| IBIS file stm32l0_71_72_73_81_82_83_lqfp64.ibs
| Created by s2ibis version 1.1 (customized version)
| North Carolina State University, ERL, 2006
[IBIS ver] 4.2
[File name] stm32l0_71_72_73_81_82_83_lqfp64.ibs
[File Rev] 1.0
[Date]  14-03-2016
[Source] Data Created at STMicroelectronics
[Notes]  File originated from ELDO simulations.
[Disclaimer]  This information is for modeling purpose only and is
   not guaranted. The information is subject to change without
   notice.
[Copyright] Copyright 2016 STMicroelectronics Inc.
|   Component stm32l0_71_72_73_81_82_83_lqfp64
[Component] stm32l0_71_72_73_81_82_83_lqfp64
[Manufacturer] STMicroelectronics
[Package]
| variable   typ   min   max
R_pkg   0.0   0.0   0.0
L_pkg   0.0H   0.0H   0.0H
C_pkg   0.0F   0.0F   0.0F
[Pin]  signal_name   model_name   R_pin   L_pin   C_pin
1 VLCD POWER   68.980E-3   4.220E-9   120.000E-15
2 PC13 io8p_wsudq_ls_ft_v33   63.756E-3   3.679E-9   93.469E-15
3 PC14-OSC32_IN io8p_wsudq_ls_ft_v33   59.336E-3   3.221E-9   71.020E-15
4 PC15-OSC32_OUT io8p_sudq_ls_tc_esdft 55.719E-3   2.846E-9   52.653E-15
5 PH0-OSC_IN io8p_sudq_ls_tc_esdft   52.907E-3   2.555E-9   38.367E-15
6 PH1-OSC_OUT io8p_sudq_ls_tc_esdft   50.897E-3   2.347E-9   28.163E-15
7 NRST ioreset_ft_v33   49.692E-3   2.222E-9   22.041E-15
8 PC0 io8p_sudq_lcd4_i2cin_ls_ft   49.290E-3   2.180E-9   20.000E-15
9 PC1 io8p_sudq_lcd4_i2cin_ls_ft   49.290E-3   2.180E-9   20.000E-15
10 PC2 io8p_wsudq_lcd4_ls_ft   49.692E-3   2.222E-9   22.041E-15
11 PC3 io8p_wsudq_lcd4_ls_ft   50.897E-3   2.347E-9   28.163E-15
12 VSSA GND   52.907E-3   2.555E-9   38.367E-15
13 VDDA POWER   55.719E-3   2.846E-9   52.653E-15
14 PA0 io8p_wsudq_ls_ft_v33   59.336E-3   3.221E-9   71.020E-15
15 PA1 io8p_wsudq_lcd4_ls_ft  63.756E-3   3.679E-9   93.469E-15
16 PA2 io8p_wsudq_lcd4_ls_ft  68.980E-3   4.220E-9   120.000E-15
17 PA3 io8p_wsudq_lcd4_ls_ft  68.980E-3   4.220E-9   120.000E-15
18 VSS GND   63.756E-3   3.679E-9   93.469E-15
19 VDD POWER   59.336E-3   3.221E-9   71.020E-15
20 PA4 io8p_wsudq_i2cin_ls_ft 55.719E-3   2.846E-9   52.653E-15
21 PA5 io8p_wsudq_i2cin_ls_ft 52.907E-3   2.555E-9   38.367E-15
22 PA6 io8p_wsudq_lcd4_ls_ft  50.897E-3   2.347E-9   28.163E-15
23 PA7 io8p_wsudq_lcd4_ls_ft  49.692E-3   2.222E-9   22.041E-15
24 PC4 io8p_wsudq_lcd4_ls_ft  49.290E-3   2.180E-9   20.000E-15
25 PC5 io8p_wsudq_lcd4_ls_ft  49.290E-3   2.180E-9   20.000E-15
26 PB0 io8p_wsudq_lcd4_ls_ft  49.692E-3   2.222E-9   22.041E-15
27 PB1 io8p_wsudq_lcd4_ls_ft  50.897E-3   2.347E-9   28.163E-15
28 PB2 io8p_wsudq_lcd4_ls_ft  52.907E-3   2.555E-9   38.367E-15
29 PB10 io8p_sudq_lcd4_i2cin_ls_ft   55.719E-3   2.846E-9   52.653E-15
30 PB11 io8p_sudq_lcd4_i2cin_ls_ft   59.336E-3   3.221E-9   71.020E-15
31 VSS GND   63.756E-3   3.679E-9   93.469E-15
32 VDD POWER   68.980E-3   4.220E-9   120.000E-15
33 PB12 io8p_wsudq_lcd4_ls_ft 68.980E-3   4.220E-9   120.000E-15
34 PB13 io8p_sudq_lcd4_i2cin_ls_ft   63.756E-3   3.679E-9   93.469E-15
35 PB14 io8p_sudq_lcd4_i2cin_ls_ft   59.336E-3   3.221E-9   71.020E-15
36 PB15 io8p_wsudq_lcd4_ls_ft   55.719E-3   2.846E-9   52.653E-15
37 PC6 io8p_wsudq_lcd4_ls_ft   52.907E-3   2.555E-9   38.367E-15
38 PC7 io8p_wsudq_lcd4_ls_ft   50.897E-3   2.347E-9   28.163E-15
39 PC8 io8p_wsudq_lcd4_ls_ft   49.692E-3   2.222E-9   22.041E-15
40 PC9 io8p_sudq_lcd4_i2cin_ls_ft   49.290E-3   2.180E-9   20.000E-15
41 PA8 io8p_sudq_lcd4_i2cin_ls_ft   49.290E-3   2.180E-9   20.000E-15
42 PA9 io8p_sudq_lcd4_i2cin_ls_ft   49.692E-3   2.222E-9   22.041E-15
43 PA10 io8p_sudq_lcd4_i2cin_ls_ft   50.897E-3   2.347E-9   28.163E-15
44 PA11 io8usb_ls_ft   52.907E-3   2.555E-9   38.367E-15
45 PA12 io8usb_ls_ft   55.719E-3   2.846E-9   52.653E-15
46 PA13 io8p_sudq_ls_ft   59.336E-3   3.221E-9   71.020E-15
47 VSS GND   63.756E-3   3.679E-9   93.469E-15
48 VDD_USB POWER   68.980E-3   4.220E-9   120.000E-15
49 PA14 io8p_sudq_ls_ft   68.980E-3   4.220E-9   120.000E-15
50 PA15 io8p_wsudq_lcd4_ls_ft   63.756E-3   3.679E-9   93.469E-15
51 PC10 io8p_wsudq_lcd4_ls_ft   59.336E-3   3.221E-9   71.020E-15
52 PC11 io8p_wsudq_lcd4_ls_ft   55.719E-3   2.846E-9   52.653E-15
53 PC12 io8p_wsudq_lcd4_ls_ft   52.907E-3   2.555E-9   38.367E-15
54 PD2 io8p_wsudq_lcd4_ls_ft   50.897E-3   2.347E-9   28.163E-15
55 PB3 io8p_wsudq_lcd4_ls_ft   49.692E-3   2.222E-9   22.041E-15
56 PB4 io8p_sudq_lcd4_i2cin_ls_ft 49.290E-3   2.180E-9   20.000E-15
57 PB5 io8p_wsudq_lcd4_ls_ft   49.290E-3   2.180E-9   20.000E-15
58 PB6 io8p_wsudq_i2cin_ls_ft   49.692E-3   2.222E-9   22.041E-15
59 PB7 io8p_wsudq_i2cin_ls_ft   50.897E-3   2.347E-9   28.163E-15
60 BOOT0 vpp_test_hv  52.907E-3   2.555E-9   38.367E-15
61 PB8 io8p_sudq_lcd4_i2cin_ls_ft   55.719E-3   2.846E-9   52.653E-15
62 PB9 io8p_sudq_lcd4_i2cin_ls_ft   59.336E-3   3.221E-9   71.020E-15
63 VSS GND   63.756E-3   3.679E-9   93.469E-15
64 VDD POWER   68.980E-3   4.220E-9   120.000E-15
[Model Selector] io8p_sudq_ls_ft
io8p00_sudq_ls_ft_pd_lv  "SPEED00 1P8V, PD=40kOhm"
io8p00_sudq_ls_ft_pu_lv  "SPEED00 1P8V, PU=40kOhm"
io8p00_sudq_ls_ft_lv  "SPEED00 1P8V"
io8p01_sudq_ls_ft_pd_lv  "SPEED01 1P8V, PD=40kOhm"
io8p01_sudq_ls_ft_pu_lv  "SPEED01 1P8V, PU=40kOhm"
io8p01_sudq_ls_ft_lv  "SPEED01 1P8V"
io8p10_sudq_ls_ft_pd_lv  "SPEED10 1P8V, PD=40kOhm"
io8p10_sudq_ls_ft_pu_lv  "SPEED10 1P8V, PU=40kOhm"
io8p10_sudq_ls_ft_lv  "SPEED10 1P8V"
io8p11_sudq_ls_ft_pd_lv  "SPEED11 1P8V, PD=40kOhm"
io8p11_sudq_ls_ft_pu_lv  "SPEED11 1P8V, PU=40kOhm"
io8p11_sudq_ls_ft_lv  "SPEED11 1P8V"
io8p00_sudq_ls_ft_pd  "SPEED00, PD=40kOhm"
io8p00_sudq_ls_ft_pu  "SPEED00, PU=40kOhm"
io8p00_sudq_ls_ft  "SPEED00"
io8p01_sudq_ls_ft_pd  "SPEED01, PD=40kOhm"
io8p01_sudq_ls_ft_pu  "SPEED01, PU=40kOhm"
io8p01_sudq_ls_ft  "SPEED01"
io8p10_sudq_ls_ft_pd  "SPEED10, PD=40kOhm"
io8p10_sudq_ls_ft_pu  "SPEED10, PU=40kOhm"
io8p10_sudq_ls_ft  "SPEED10"
io8p11_sudq_ls_ft_pd  "SPEED11, PD=40kOhm"
io8p11_sudq_ls_ft_pu  "SPEED11, PU=40kOhm"
io8p11_sudq_ls_ft  "SPEED11"
[Model Selector] io8p_sudq_ls_tc_esdft
io8p00_sudq_ls_tc_esdft_pd_lv  "SPEED00 1P8V, PD=40kOhm"
io8p00_sudq_ls_tc_esdft_pu_lv  "SPEED00 1P8V, PU=40kOhm"
io8p00_sudq_ls_tc_esdft_lv  "SPEED00 1P8V"
io8p01_sudq_ls_tc_esdft_pd_lv  "SPEED01 1P8V, PD=40kOhm"
io8p01_sudq_ls_tc_esdft_pu_lv  "SPEED01 1P8V, PU=40kOhm"
io8p01_sudq_ls_tc_esdft_lv  "SPEED01 1P8V"
io8p10_sudq_ls_tc_esdft_pd_lv  "SPEED10 1P8V, PD=40kOhm"
io8p10_sudq_ls_tc_esdft_pu_lv  "SPEED10 1P8V, PU=40kOhm"
io8p10_sudq_ls_tc_esdft_lv  "SPEED10 1P8V"
io8p11_sudq_ls_tc_esdft_pd_lv  "SPEED11 1P8V, PD=40kOhm"
io8p11_sudq_ls_tc_esdft_pu_lv  "SPEED11 1P8V, PU=40kOhm"
io8p11_sudq_ls_tc_esdft_lv  "SPEED11 1P8V"
io8p00_sudq_ls_tc_esdft_pd  "SPEED00, PD=40kOhm"
io8p00_sudq_ls_tc_esdft_pu  "SPEED00, PU=40kOhm"
io8p00_sudq_ls_tc_esdft  "SPEED00"
io8p01_sudq_ls_tc_esdft_pd  "SPEED01, PD=40kOhm"
io8p01_sudq_ls_tc_esdft_pu  "SPEED01, PU=40kOhm"
io8p01_sudq_ls_tc_esdft  "SPEED01"
io8p10_sudq_ls_tc_esdft_pd  "SPEED10, PD=40kOhm"
io8p10_sudq_ls_tc_esdft_pu  "SPEED10, PU=40kOhm"
io8p10_sudq_ls_tc_esdft  "SPEED10"
io8p11_sudq_ls_tc_esdft_pd  "SPEED11, PD=40kOhm"
io8p11_sudq_ls_tc_esdft_pu  "SPEED11, PU=40kOhm"
io8p11_sudq_ls_tc_esdft  "SPEED11"
[Model Selector] io8p_wsudq_i2cin_ls_ft
io8p00_wsudq_i2cin_ls_ft_pd_lv  "SPEED00 1P8V, PD=40kOhm"
io8p00_wsudq_i2cin_ls_ft_pu_lv  "SPEED00 1P8V, PU=40kOhm"
io8p00_wsudq_i2cin_ls_ft_lv  "SPEED00 1P8V"
io8p01_wsudq_i2cin_ls_ft_pd_lv  "SPEED01 1P8V, PD=40kOhm"
io8p01_wsudq_i2cin_ls_ft_pu_lv  "SPEED01 1P8V, PU=40kOhm"
io8p01_wsudq_i2cin_ls_ft_lv  "SPEED01 1P8V"
io8p10_wsudq_i2cin_ls_ft_pd_lv  "SPEED10 1P8V, PD=40kOhm"
io8p10_wsudq_i2cin_ls_ft_pu_lv  "SPEED10 1P8V, PU=40kOhm"
io8p10_wsudq_i2cin_ls_ft_lv  "SPEED10 1P8V"
io8p11_wsudq_i2cin_ls_ft_pd_lv  "SPEED11 1P8V, PD=40kOhm"
io8p11_wsudq_i2cin_ls_ft_pu_lv  "SPEED11 1P8V, PU=40kOhm"
io8p11_wsudq_i2cin_ls_ft_lv  "SPEED11 1P8V"
io8p00_wsudq_i2cin_ls_ft_pd  "SPEED00, PD=40kOhm"
io8p00_wsudq_i2cin_ls_ft_pu  "SPEED00, PU=40kOhm"
io8p00_wsudq_i2cin_ls_ft  "SPEED00"
io8p01_wsudq_i2cin_ls_ft_pd  "SPEED01, PD=40kOhm"
io8p01_wsudq_i2cin_ls_ft_pu  "SPEED01, PU=40kOhm"
io8p01_wsudq_i2cin_ls_ft  "SPEED01"
io8p10_wsudq_i2cin_ls_ft_pd  "SPEED10, PD=40kOhm"
io8p10_wsudq_i2cin_ls_ft_pu  "SPEED10, PU=40kOhm"
io8p10_wsudq_i2cin_ls_ft  "SPEED10"
io8p11_wsudq_i2cin_ls_ft_pd  "SPEED11, PD=40kOhm"
io8p11_wsudq_i2cin_ls_ft_pu  "SPEED11, PU=40kOhm"
io8p11_wsudq_i2cin_ls_ft  "SPEED11"
[Model Selector] io8p_wsudq_lcd4_ls_ft
io8p00_wsudq_lcd4_ls_ft_pd_lv  "SPEED00 1P8V, PD=40kOhm"
io8p00_wsudq_lcd4_ls_ft_pu_lv  "SPEED00 1P8V, PU=40kOhm"
io8p00_wsudq_lcd4_ls_ft_lv  "SPEED00 1P8V"
io8p01_wsudq_lcd4_ls_ft_pd_lv  "SPEED01 1P8V, PD=40kOhm"
io8p01_wsudq_lcd4_ls_ft_pu_lv  "SPEED01 1P8V, PU=40kOhm"
io8p01_wsudq_lcd4_ls_ft_lv  "SPEED01 1P8V"
io8p10_wsudq_lcd4_ls_ft_pd_lv  "SPEED10 1P8V, PD=40kOhm"
io8p10_wsudq_lcd4_ls_ft_pu_lv  "SPEED10 1P8V, PU=40kOhm"
io8p10_wsudq_lcd4_ls_ft_lv  "SPEED10 1P8V"
io8p11_wsudq_lcd4_ls_ft_pd_lv  "SPEED11 1P8V, PD=40kOhm"
io8p11_wsudq_lcd4_ls_ft_pu_lv  "SPEED11 1P8V, PU=40kOhm"
io8p11_wsudq_lcd4_ls_ft_lv  "SPEED11 1P8V"
io8p00_wsudq_lcd4_ls_ft_pd  "SPEED00, PD=40kOhm"
io8p00_wsudq_lcd4_ls_ft_pu  "SPEED00, PU=40kOhm"
io8p00_wsudq_lcd4_ls_ft  "SPEED00"
io8p01_wsudq_lcd4_ls_ft_pd  "SPEED01, PD=40kOhm"
io8p01_wsudq_lcd4_ls_ft_pu  "SPEED01, PU=40kOhm"
io8p01_wsudq_lcd4_ls_ft  "SPEED01"
io8p10_wsudq_lcd4_ls_ft_pd  "SPEED10, PD=40kOhm"
io8p10_wsudq_lcd4_ls_ft_pu  "SPEED10, PU=40kOhm"
io8p10_wsudq_lcd4_ls_ft  "SPEED10"
io8p11_wsudq_lcd4_ls_ft_pd  "SPEED11, PD=40kOhm"
io8p11_wsudq_lcd4_ls_ft_pu  "SPEED11, PU=40kOhm"
io8p11_wsudq_lcd4_ls_ft  "SPEED11"
[Model Selector] io8p_wsudq_ls_ft_v33
io8p00_wsudq_ls_ft_v33_pd_lv  "SPEED00 1P8V, PD=40kOhm"
io8p00_wsudq_ls_ft_v33_pu_lv  "SPEED00 1P8V, PU=40kOhm"
io8p00_wsudq_ls_ft_v33_lv  "SPEED00 1P8V"
io8p01_wsudq_ls_ft_v33_pd_lv  "SPEED01 1P8V, PD=40kOhm"
io8p01_wsudq_ls_ft_v33_pu_lv  "SPEED01 1P8V, PU=40kOhm"
io8p01_wsudq_ls_ft_v33_lv  "SPEED01 1P8V"
io8p10_wsudq_ls_ft_v33_pd_lv  "SPEED10 1P8V, PD=40kOhm"
io8p10_wsudq_ls_ft_v33_pu_lv  "SPEED10 1P8V, PU=40kOhm"
io8p10_wsudq_ls_ft_v33_lv  "SPEED10 1P8V"
io8p11_wsudq_ls_ft_v33_pd_lv  "SPEED11 1P8V, PD=40kOhm"
io8p11_wsudq_ls_ft_v33_pu_lv  "SPEED11 1P8V, PU=40kOhm"
io8p11_wsudq_ls_ft_v33_lv  "SPEED11 1P8V"
io8p00_wsudq_ls_ft_v33_pd  "SPEED00, PD=40kOhm"
io8p00_wsudq_ls_ft_v33_pu  "SPEED00, PU=40kOhm"
io8p00_wsudq_ls_ft_v33  "SPEED00"
io8p01_wsudq_ls_ft_v33_pd  "SPEED01, PD=40kOhm"
io8p01_wsudq_ls_ft_v33_pu  "SPEED01, PU=40kOhm"
io8p01_wsudq_ls_ft_v33  "SPEED01"
io8p10_wsudq_ls_ft_v33_pd  "SPEED10, PD=40kOhm"
io8p10_wsudq_ls_ft_v33_pu  "SPEED10, PU=40kOhm"
io8p10_wsudq_ls_ft_v33  "SPEED10"
io8p11_wsudq_ls_ft_v33_pd  "SPEED11, PD=40kOhm"
io8p11_wsudq_ls_ft_v33_pu  "SPEED11, PU=40kOhm"
io8p11_wsudq_ls_ft_v33  "SPEED11"
[Model Selector] vpp_test_hv
vpp_test_hv_2p4  "Input Buffer 1P65V"
vpp_test_hv_3p3  "Input Buffer"
[Model Selector] io8usb_ls_ft
io8usb_ls_ft_dpdn_pu  "HS USB DP/DN IO + PU=1.2kOhm"
io8usb_ls_ft_dpdn  "HS USB DP/DN IO"
io8p00_ls_ft_pd_lv  "SPEED00 1P8V, PD=40kOhm"
io8p00_ls_ft_pu_lv  "SPEED00 1P8V, PU=40kOhm"
io8p00_ls_ft_lv  "SPEED00 1P8V"
io8p01_ls_ft_pd_lv  "SPEED01 1P8V, PD=40kOhm"
io8p01_ls_ft_pu_lv  "SPEED01 1P8V, PU=40kOhm"
io8p01_ls_ft_lv  "SPEED01 1P8V"
io8p10_ls_ft_pd_lv  "SPEED10 1P8V, PD=40kOhm"
io8p10_ls_ft_pu_lv  "SPEED10 1P8V, PU=40kOhm"
io8p10_ls_ft_lv  "SPEED10 1P8V"
io8p11_ls_ft_pd_lv  "SPEED11 1P8V, PD=40kOhm"
io8p11_ls_ft_pu_lv  "SPEED11 1P8V, PU=40kOhm"
io8p11_ls_ft_lv  "SPEED11 1P8V"
io8p00_ls_ft_pd  "SPEED00, PD=40kOhm"
io8p00_ls_ft_pu  "SPEED00, PU=40kOhm"
io8p00_ls_ft  "SPEED00"
io8p01_ls_ft_pd  "SPEED01, PD=40kOhm"
io8p01_ls_ft_pu  "SPEED01, PU=40kOhm"
io8p01_ls_ft  "SPEED01"
io8p10_ls_ft_pd  "SPEED10, PD=40kOhm"
io8p10_ls_ft_pu  "SPEED10, PU=40kOhm"
io8p10_ls_ft  "SPEED10"
io8p11_ls_ft_pd  "SPEED11, PD=40kOhm"
io8p11_ls_ft_pu  "SPEED11, PU=40kOhm"
io8p11_ls_ft  "SPEED11"
[Model Selector] io8p_sudq_lcd4_i2cin_ls_ft
io8p00_sudq_lcd4_i2cin_ls_ft_pd_lv  "SPEED00 1P8V, PD=40kOhm"
io8p00_sudq_lcd4_i2cin_ls_ft_pu_lv  "SPEED00 1P8V, PU=40kOhm"
io8p00_sudq_lcd4_i2cin_ls_ft_lv  "SPEED00 1P8V"
io8p01_sudq_lcd4_i2cin_ls_ft_pd_lv  "SPEED01 1P8V, PD=40kOhm"
io8p01_sudq_lcd4_i2cin_ls_ft_pu_lv  "SPEED01 1P8V, PU=40kOhm"
io8p01_sudq_lcd4_i2cin_ls_ft_lv  "SPEED01 1P8V"
io8p10_sudq_lcd4_i2cin_ls_ft_pd_lv  "SPEED10 1P8V, PD=40kOhm"
io8p10_sudq_lcd4_i2cin_ls_ft_pu_lv  "SPEED10 1P8V, PU=40kOhm"
io8p10_sudq_lcd4_i2cin_ls_ft_lv  "SPEED10 1P8V"
io8p11_sudq_lcd4_i2cin_ls_ft_pd_lv  "SPEED11 1P8V, PD=40kOhm"
io8p11_sudq_lcd4_i2cin_ls_ft_pu_lv  "SPEED11 1P8V, PU=40kOhm"
io8p11_sudq_lcd4_i2cin_ls_ft_lv  "SPEED11 1P8V"
io8p00_sudq_lcd4_i2cin_ls_ft_pd  "SPEED00, PD=40kOhm"
io8p00_sudq_lcd4_i2cin_ls_ft_pu  "SPEED00, PU=40kOhm"
io8p00_sudq_lcd4_i2cin_ls_ft  "SPEED00"
io8p01_sudq_lcd4_i2cin_ls_ft_pd  "SPEED01, PD=40kOhm"
io8p01_sudq_lcd4_i2cin_ls_ft_pu  "SPEED01, PU=40kOhm"
io8p01_sudq_lcd4_i2cin_ls_ft  "SPEED01"
io8p10_sudq_lcd4_i2cin_ls_ft_pd  "SPEED10, PD=40kOhm"
io8p10_sudq_lcd4_i2cin_ls_ft_pu  "SPEED10, PU=40kOhm"
io8p10_sudq_lcd4_i2cin_ls_ft  "SPEED10"
io8p11_sudq_lcd4_i2cin_ls_ft_pd  "SPEED11, PD=40kOhm"
io8p11_sudq_lcd4_i2cin_ls_ft_pu  "SPEED11, PU=40kOhm"
io8p11_sudq_lcd4_i2cin_ls_ft  "SPEED11"
[Model Selector] ioreset_ft_v33
ioreset_ft_v33_pu_lv  "ioreset 1P8V + PU=40kOhm"
ioreset_ft_v33_nopu_lv  "ioreset 1P8V"
ioreset_ft_v33_pu  "ioreset + PU=40kOhm"
ioreset_ft_v33_nopu  "ioreset"
| Models and submodels in the file (176): io8p00_sudq_ls_ft_pd_lv (I/O), io8p00_sudq_ls_ft_pu_lv (I/O), io8p00_sudq_ls_ft_lv (I/O), io8p01_sudq_ls_ft_pd_lv (I/O), io8p01_sudq_ls_ft_pu_lv (I/O), io8p01_sudq_ls_ft_lv (I/O), io8p10_sudq_ls_ft_pd_lv (I/O), io8p10_sudq_ls_ft_pu_lv (I/O), io8p10_sudq_ls_ft_lv (I/O), io8p11_sudq_ls_ft_pd_lv (I/O), io8p11_sudq_ls_ft_pu_lv (I/O), io8p11_sudq_ls_ft_lv (I/O), io8p00_sudq_ls_ft_pd (I/O), io8p00_sudq_ls_ft_pu (I/O), io8p00_sudq_ls_ft (I/O), io8p01_sudq_ls_ft_pd (I/O), io8p01_sudq_ls_ft_pu (I/O), io8p01_sudq_ls_ft (I/O), io8p10_sudq_ls_ft_pd (I/O), io8p10_sudq_ls_ft_pu (I/O), io8p10_sudq_ls_ft (I/O), io8p11_sudq_ls_ft_pd (I/O), io8p11_sudq_ls_ft_pu (I/O), io8p11_sudq_ls_ft (I/O), io8p00_sudq_ls_tc_esdft_pd_lv (I/O), io8p00_sudq_ls_tc_esdft_pu_lv (I/O), io8p00_sudq_ls_tc_esdft_lv (I/O), io8p01_sudq_ls_tc_esdft_pd_lv (I/O), io8p01_sudq_ls_tc_esdft_pu_lv (I/O), io8p01_sudq_ls_tc_esdft_lv (I/O), io8p10_sudq_ls_tc_esdft_pd_lv (I/O), io8p10_sudq_ls_tc_esdft_pu_lv (I/O), io8p10_sudq_ls_tc_esdft_lv (I/O), io8p11_sudq_ls_tc_esdft_pd_lv (I/O), io8p11_sudq_ls_tc_esdft_pu_lv (I/O), io8p11_sudq_ls_tc_esdft_lv (I/O), io8p00_sudq_ls_tc_esdft_pd (I/O), io8p00_sudq_ls_tc_esdft_pu (I/O), io8p00_sudq_ls_tc_esdft (I/O), io8p01_sudq_ls_tc_esdft_pd (I/O), io8p01_sudq_ls_tc_esdft_pu (I/O), io8p01_sudq_ls_tc_esdft (I/O), io8p10_sudq_ls_tc_esdft_pd (I/O), io8p10_sudq_ls_tc_esdft_pu (I/O), io8p10_sudq_ls_tc_esdft (I/O), io8p11_sudq_ls_tc_esdft_pd (I/O), io8p11_sudq_ls_tc_esdft_pu (I/O), io8p11_sudq_ls_tc_esdft (I/O), io8p00_wsudq_i2cin_ls_ft_pd_lv (I/O), io8p00_wsudq_i2cin_ls_ft_pu_lv (I/O), io8p00_wsudq_i2cin_ls_ft_lv (I/O), io8p01_wsudq_i2cin_ls_ft_pd_lv (I/O), io8p01_wsudq_i2cin_ls_ft_pu_lv (I/O), io8p01_wsudq_i2cin_ls_ft_lv (I/O), io8p10_wsudq_i2cin_ls_ft_pd_lv (I/O), io8p10_wsudq_i2cin_ls_ft_pu_lv (I/O), io8p10_wsudq_i2cin_ls_ft_lv (I/O), io8p11_wsudq_i2cin_ls_ft_pd_lv (I/O), io8p11_wsudq_i2cin_ls_ft_pu_lv (I/O), io8p11_wsudq_i2cin_ls_ft_lv (I/O), io8p00_wsudq_i2cin_ls_ft_pd (I/O), io8p00_wsudq_i2cin_ls_ft_pu (I/O), io8p00_wsudq_i2cin_ls_ft (I/O), io8p01_wsudq_i2cin_ls_ft_pd (I/O), io8p01_wsudq_i2cin_ls_ft_pu (I/O), io8p01_wsudq_i2cin_ls_ft (I/O), io8p10_wsudq_i2cin_ls_ft_pd (I/O), io8p10_wsudq_i2cin_ls_ft_pu (I/O), io8p10_wsudq_i2cin_ls_ft (I/O), io8p11_wsudq_i2cin_ls_ft_pd (I/O), io8p11_wsudq_i2cin_ls_ft_pu (I/O), io8p11_wsudq_i2cin_ls_ft (I/O), io8p00_wsudq_lcd4_ls_ft_pd_lv (I/O), io8p00_wsudq_lcd4_ls_ft_pu_lv (I/O), io8p00_wsudq_lcd4_ls_ft_lv (I/O), io8p01_wsudq_lcd4_ls_ft_pd_lv (I/O), io8p01_wsudq_lcd4_ls_ft_pu_lv (I/O), io8p01_wsudq_lcd4_ls_ft_lv (I/O), io8p10_wsudq_lcd4_ls_ft_pd_lv (I/O), io8p10_wsudq_lcd4_ls_ft_pu_lv (I/O)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
